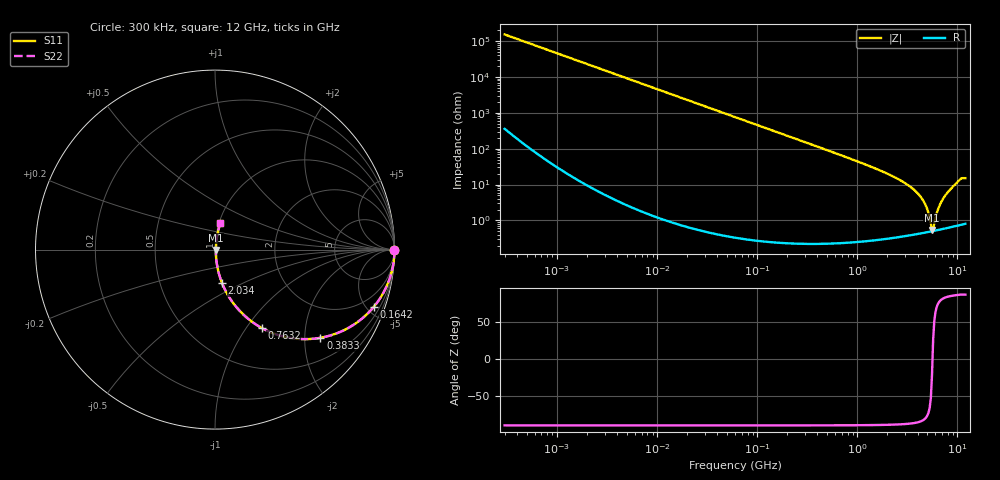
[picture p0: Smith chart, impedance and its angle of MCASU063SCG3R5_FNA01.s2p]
! MCASU063SCG3R5_FNA01  S-PARAMETER MODEL  ( General Type )
! Model Generated by TAIYO YUDEN Corporation (http://www.ty-top.com)
! Version 1.0
! TAIYO YUDEN Control No. 130801
! Copyright(c) 2013 TAIYO YUDEN CO.,LTD. All Rights Reserved.
! Product Description (link to TY-COMPAS)
! https://ds.yuden.co.jp/TYCOMPAS/or/detail?pn=MCASU063SCG3R5CFNA01&u=M
! Products Name : Multilayer Ceramic Capacitors
! Characteristics :
!  Capacitance : 3.5 pF , Rated Voltage : 50V , TCC : CG / C0G
!  Case Size : 0.6 x 0.3 / 0.024 x 0.012 [mm/inch] , Thickness : 0.3 / 0.012 [mm/inch]
!  (Conditions: Temperature = 25 degC , DC Bias Current/Voltage = 0A / 0V)
! External Node Assignments :
!  1  o---| |---o  2
! GND o---------o GND
! Frequency Range : 0.3MHz  -  12000MHz  [ 401 STEP ]
# MHz S RI R 50
! Freq[MHz].  S11 Real  S11 Imag  S21 Real  S21 Imag  S12 Real  S12 Imag  S22 Real  S22 Imag
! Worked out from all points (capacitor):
!   401 points, 300 kHz to 12 GHz, reference 50 ohm
!   read as one part in series: C = 3.47 pF near 316.3 kHz
!   lowest |Z| = 540 mohm at 5.566 GHz (marker M1)
!   series resonance near 5.634 GHz, so ESL is about 230 pH
!   S11 on the Smith chart (normalised r, x): 300 kHz: open; 164.2 MHz: 1.00, -5.59; 383.3 MHz: 1.00, -2.38; 763.2 MHz: 1.00, -1.18; 2.034 GHz: 1.01, -0.39; 12 GHz: 1.02, +0.30
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0.3  1 -0.000654  1.96e-06 0.000654  1.96e-06 0.000654  1 -0.000654
1.769972  1 -0.00386  1.66e-05 0.00386  1.66e-05 0.00386  1 -0.00386
10.44266  0.9995 -0.0227  0.000523 0.0227  0.000523 0.0227  0.9995 -0.0227
60  0.9831 -0.1285  0.0169 0.1285  0.0169 0.1285  0.9831 -0.1285
164.1901  0.8862 -0.3172  0.1138 0.3172  0.1138 0.3172  0.8862 -0.3172
353.9943  0.625 -0.4833  0.375 0.4833  0.375 0.4833  0.625 -0.4833
383.2761  0.5868 -0.4915  0.4132 0.4915  0.4132 0.4915  0.5868 -0.4915
763.2128  0.2594 -0.4363  0.7406 0.4363  0.7406 0.4363  0.2594 -0.4363
1197.383  0.12 -0.3214  0.88 0.3214  0.88 0.3214  0.12 -0.3214
2033.931  0.0399 -0.188  0.9601 0.188  0.9601 0.188  0.0399 -0.188
2088.533  0.0376 -0.182  0.9624 0.182  0.9624 0.182  0.0376 -0.182
3190.978  0.0131 -0.0962  0.9869 0.0962  0.9869 0.0962  0.0131 -0.0962
4158.869  0.00677 -0.0499  0.9932 0.0499  0.9932 0.0499  0.00677 -0.0499
4875.354  0.0052 -0.0237  0.9948 0.0237  0.9948 0.0237  0.0052 -0.0237
5420.343  0.00495 -0.00652  0.995 0.00652  0.995 0.00652  0.00495 -0.00652
5565.855  0.00499 -0.00202  0.995 0.00202  0.995 0.00202  0.00499 -0.00202
5715.274  0.00506 0.00243  0.9949 -0.00243  0.9949 -0.00243  0.00506 0.00243
5868.704  0.00517 0.00641  0.9948 -0.00641  0.9948 -0.00641  0.00517 0.00641
6524.734  0.00597 0.0227  0.994 -0.0227  0.994 -0.0227  0.00597 0.0227
7448.838  0.00805 0.0462  0.9919 -0.0462  0.9919 -0.0462  0.00805 0.0462
10511.28  0.0248 0.1303  0.9752 -0.1303  0.9752 -0.1303  0.0248 0.1303
12000  0.0298 0.1454  0.9702 -0.1454  0.9702 -0.1454  0.0298 0.1454
